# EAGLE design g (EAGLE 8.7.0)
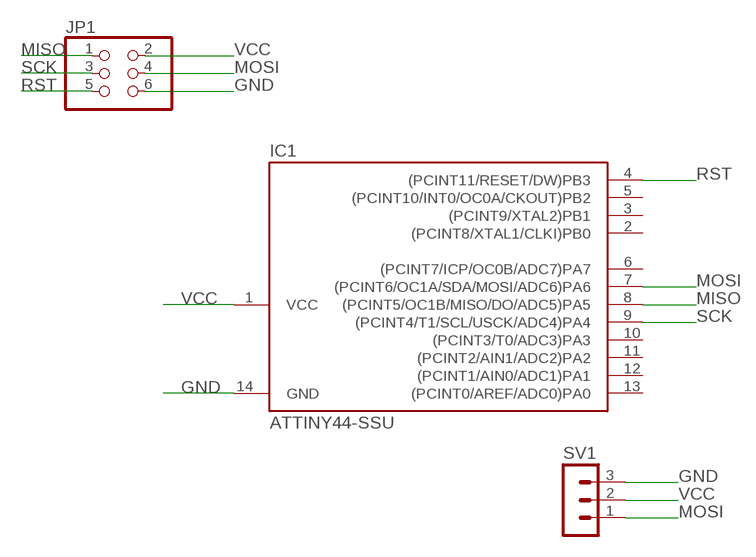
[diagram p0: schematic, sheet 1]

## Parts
IC1  ATTINY44-SSU  [SOIC14]
JP1  PINHD-2X3-SMD  [2X03SMD]
SV1  MA03-1  [MA03-1]

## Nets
GND: IC1.14(GND) JP1.6 SV1.3
MISO: IC1.8((PCINT5/OC1B/MISO/DO/ADC5)PA5) JP1.1
MOSI: IC1.7((PCINT6/OC1A/SDA/MOSI/ADC6)PA6) JP1.4 SV1.1
RST: IC1.4((PCINT11/RESET/DW)PB3) JP1.5
SCK: IC1.9((PCINT4/T1/SCL/USCK/ADC4)PA4) JP1.3
VCC: IC1.1(VCC) JP1.2 SV1.2
Unconnected: IC1.2((PCINT8/XTAL1/CLKI)PB0) IC1.3((PCINT9/XTAL2)PB1) IC1.5((PCINT10/INT0/OC0A/CKOUT)PB2) IC1.6((PCINT7/ICP/OC0B/ADC7)PA7) IC1.10((PCINT3/T0/ADC3)PA3) IC1.11((PCINT2/AIN1/ADC2)PA2) IC1.12((PCINT1/AIN0/ADC1)PA1) IC1.13((PCINT0/AREF/ADC0)PA0)

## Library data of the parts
IC1 = fab:ATTINY44
JP1 = fab:PINHD-2X3-SMD: PIN HEADER
SV1 = con-lstb:MA03-1: PIN HEADER; OC_FARNELL: unknown; OC_NEWARK: unknown

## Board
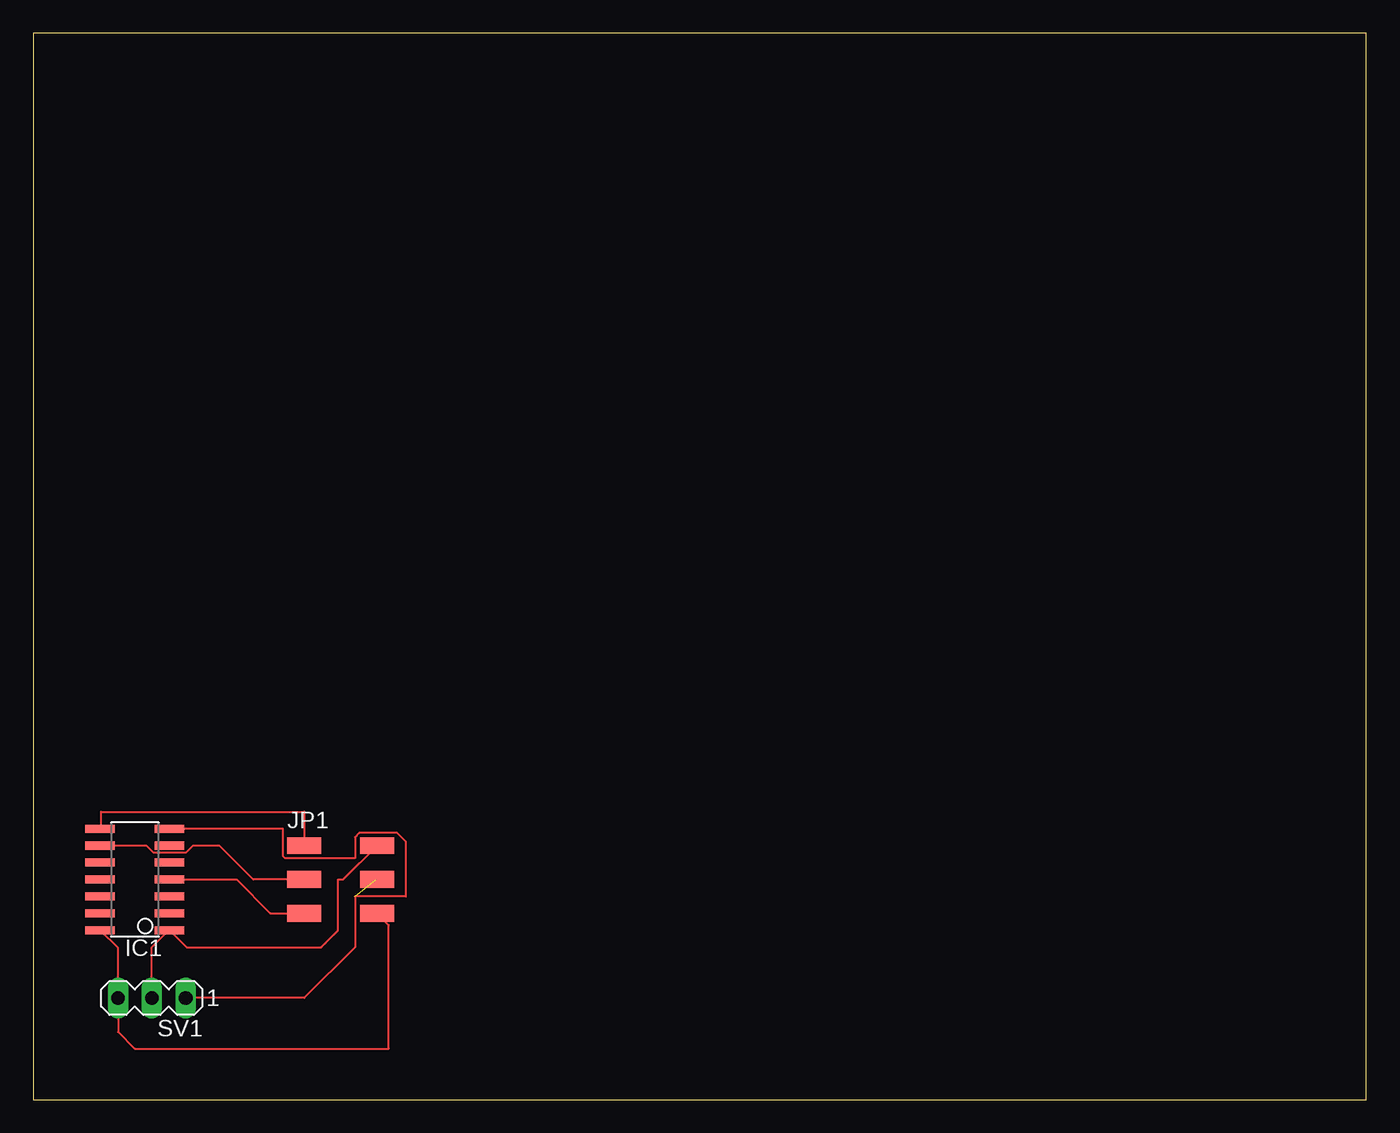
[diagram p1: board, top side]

Size 100 x 80 mm. Coordinates in mm from the lower left corner, seen from the top.
Outline: 0,0 100,0 100,80 0,80 0,0
Copper layers (1*16): Top 0.035mm / dielectric 1.5mm / Bottom 0.035mm
Design rules "default": minimum track width 6mil, minimum drill 0.35mm, track to track 6mil, track to pad 6mil, pad to pad 6mil, via to via 6mil, smd to smd 6mil, copper to edge 40mil, drill to drill 6mil, minimum pad ring 10mil, minimum via ring 8mil, stop-mask expansion 4mil, vias tented up to drill 0mil, thermal gap 10mil

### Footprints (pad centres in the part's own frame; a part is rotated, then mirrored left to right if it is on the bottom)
SOIC14 = smd 0.61 x 2.21: 1 -3.81,-2.603; 2 -2.54,-2.603; 3 -1.27,-2.603; 4 0,-2.603; 5 1.27,-2.603; 6 2.54,-2.603; 7 3.81,-2.603; 8 3.81,2.603; 9 2.54,2.603; 10 1.27,2.603; 11 0,2.603; 12 -1.27,2.603; 13 -2.54,2.603; 14 -3.81,2.603
2X03SMD = smd 2.54 x 1.27: 1 -2.54,2.54; 2 2.92,2.54; 3 -2.54,0; 4 2.92,0; 5 -2.54,-2.54; 6 2.92,-2.54
MA03-1 = drill 1.016 long: 1 -2.54,0; 2 0,0; 3 2.54,0

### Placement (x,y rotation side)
IC1  7.62,16.51 90 top
JP1  22.86,16.51 0 top
SV1  8.89,7.62 180 top

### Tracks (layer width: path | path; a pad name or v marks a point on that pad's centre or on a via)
GND
  Top 0.152: 5.08,12.7 IC1.14 6.35,11.37 SV1.3 6.35,5.08 7.62,3.81 26.67,3.81 26.67,13.08 JP1.6 25.72,13.97
MISO
  Top 0.152: IC1.8 5.08,20.38 5.08,21.59 20.32,21.59 JP1.1
MOSI  (1 unrouted)
  Top 0.152: IC1.7 18.73,20.32 18.73,18.26 18.89,18.1 24.13,18.1 24.13,19.68 24.45,20 27.3,20 27.94,19.37 27.94,15.24 24.13,15.24 24.13,11.43 20.32,7.62 SV1.1 | 25.88,16.51 JP1.4 25.72,16.51
RST
  Top 0.152: JP1.5 17.78,13.97 15.24,16.51 IC1.4
SCK
  Top 0.152: JP1.3 16.51,16.51 13.97,19.05 11.96,19.05 11.42,18.52 9.02,18.52 8.49,19.05 IC1.9
VCC
  Top 0.152: SV1.2 8.89,11.43 10.16,12.7 IC1.1 11.49,11.43 21.59,11.43 22.86,12.7 22.86,16.51 23.24,16.51 JP1.2 25.72,19.05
